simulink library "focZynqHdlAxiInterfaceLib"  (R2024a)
settings: Solver=VariableStepAuto  StartTime=0.0  StopTime=10.0  RelTol=1e-3
undefined symbols (not defined in the file or in its folder): AXI4, hex2dec, Lite
libraries: axiinterfacelib x14

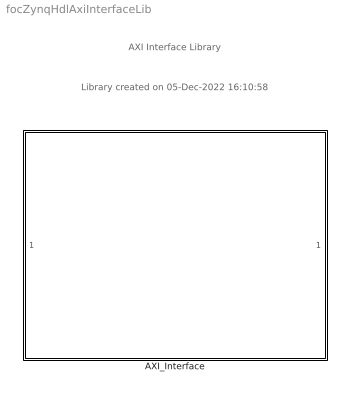
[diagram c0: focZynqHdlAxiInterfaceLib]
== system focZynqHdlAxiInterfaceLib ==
  note: AXI Interface Library
  note: Library created on 05-Dec-2022 16:10:58
  AXI_Interface : Subsystem  TreatAsAtomicUnit=on  mask(AXI4-Lite/AXI4 Interface){}
      mask help: This is an automatically generated subsystem block. This contains the AXI interface blocks that communicate with the focZynqHd_ip IPCore generated from focZynqHdl subsystem.

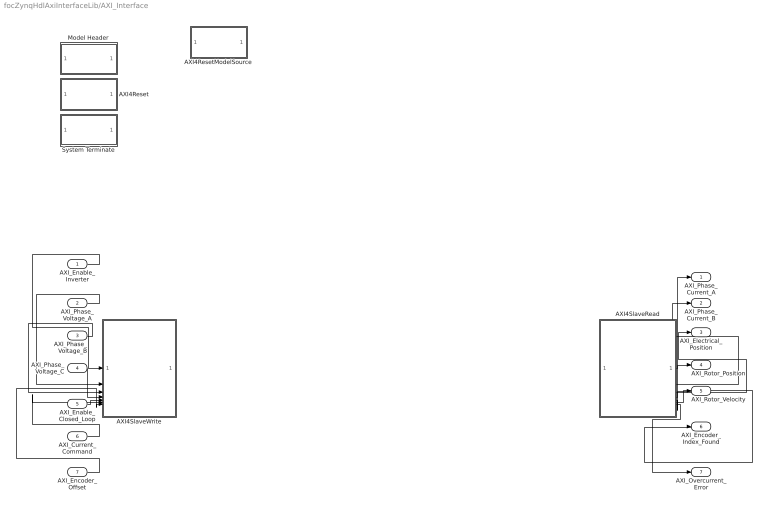
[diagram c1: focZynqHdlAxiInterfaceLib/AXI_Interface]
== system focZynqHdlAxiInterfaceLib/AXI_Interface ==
  AXI_Enable_Inverter : Inport
  AXI_Phase_Voltage_A : Inport  Port=2
  AXI_Phase_Voltage_B : Inport  Port=3
  AXI_Phase_Voltage_C : Inport  Port=4
  AXI_Enable_Closed_Loop : Inport  Port=5
  AXI_Current_Command : Inport  Port=6
  AXI_Encoder_Offset : Inport  Port=7
  AXI4Reset : Subsystem  mask(System Start){ShowInLibBrowser=0}
      mask prompts: ShowInLibBrowser "Simulink:masks:CustCodeMaskParam1_MP"
  AXI4ResetModelSource : Subsystem  mask(Model Source){ShowInLibBrowser=0}
      mask prompts: ShowInLibBrowser "Simulink:masks:CustCodeMaskParam1_MP"
  AXI4SlaveRead : Subsystem  Priority=10
  AXI4SlaveWrite : Subsystem  Priority=1
  Model Header : Subsystem  mask(Model Header){ShowInLibBrowser=0}
      mask prompts: ShowInLibBrowser "Simulink:masks:CustCodeMaskParam1_MP"
  System Terminate : Subsystem  mask(System Terminate){ShowInLibBrowser=0}
      mask prompts: ShowInLibBrowser "Simulink:masks:CustCodeMaskParam1_MP"
  AXI_Phase_Current_A : Outport  VectorParamsAs1DForOutWhenUnconnected=off
  AXI_Phase_Current_B : Outport  Port=2  VectorParamsAs1DForOutWhenUnconnected=off
  AXI_Electrical_Position : Outport  Port=3  VectorParamsAs1DForOutWhenUnconnected=off
  AXI_Rotor_Position : Outport  Port=4  VectorParamsAs1DForOutWhenUnconnected=off
  AXI_Rotor_Velocity : Outport  Port=5  VectorParamsAs1DForOutWhenUnconnected=off
  AXI_Encoder_Index_Found : Outport  Port=6  VectorParamsAs1DForOutWhenUnconnected=off
  AXI_Overcurrent_Error : Outport  Port=7  VectorParamsAs1DForOutWhenUnconnected=off
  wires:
  AXI4SlaveRead/7(AXI_Overcurrent_Error) -> AXI_Overcurrent_Error/1
  AXI4SlaveRead/6(AXI_Encoder_Index_Found) -> AXI_Encoder_Index_Found/1
  AXI4SlaveRead/5(AXI_Rotor_Velocity) -> AXI_Rotor_Velocity/1
  AXI4SlaveRead/4(AXI_Rotor_Position) -> AXI_Rotor_Position/1
  AXI4SlaveRead/3(AXI_Electrical_Position) -> AXI_Electrical_Position/1
  AXI4SlaveRead/2(AXI_Phase_Current_B) -> AXI_Phase_Current_B/1
  AXI4SlaveRead/1(AXI_Phase_Current_A) -> AXI_Phase_Current_A/1
  AXI_Encoder_Offset/1 -> AXI4SlaveWrite/7(AXI_Encoder_Offset)
  AXI_Current_Command/1 -> AXI4SlaveWrite/6(AXI_Current_Command)
  AXI_Enable_Closed_Loop/1 -> AXI4SlaveWrite/5(AXI_Enable_Closed_Loop)
  AXI_Phase_Voltage_C/1 -> AXI4SlaveWrite/4(AXI_Phase_Voltage_C)
  AXI_Phase_Voltage_B/1 -> AXI4SlaveWrite/3(AXI_Phase_Voltage_B)
  AXI_Phase_Voltage_A/1 -> AXI4SlaveWrite/2(AXI_Phase_Voltage_A)
  AXI_Enable_Inverter/1 -> AXI4SlaveWrite/1(AXI_Enable_Inverter)

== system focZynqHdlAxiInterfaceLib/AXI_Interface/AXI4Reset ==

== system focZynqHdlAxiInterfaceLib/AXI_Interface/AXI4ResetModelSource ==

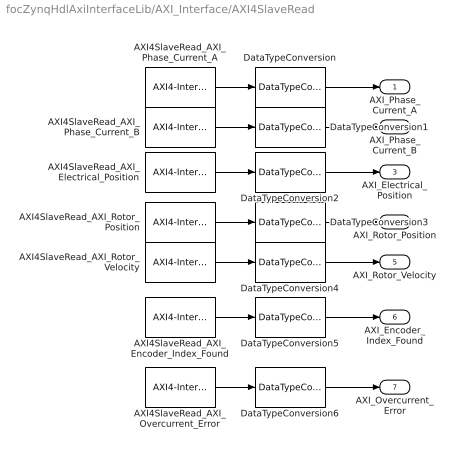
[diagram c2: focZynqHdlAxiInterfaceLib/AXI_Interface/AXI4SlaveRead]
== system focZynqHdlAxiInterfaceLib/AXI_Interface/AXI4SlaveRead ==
  AXI4SlaveRead_AXI_Electrical_Position : axiinterfacelib/AXI4-Interface Read  Priority=5  AXIInterfaceType=AXI4-Lite  DeviceName=/dev/mwipcore  RegisterOffset=hex2dec('124')  DataLength=1  DataType=uint32  SampleTime=-1  blockPlatform=ZYNQ  SimulateUsing=Interpreted Execution
  AXI4SlaveRead_AXI_Encoder_Index_Found : axiinterfacelib/AXI4-Interface Read  Priority=8  AXIInterfaceType=AXI4-Lite  DeviceName=/dev/mwipcore  RegisterOffset=hex2dec('130')  DataLength=1  DataType=uint32  SampleTime=-1  blockPlatform=ZYNQ  SimulateUsing=Interpreted Execution
  AXI4SlaveRead_AXI_Overcurrent_Error : axiinterfacelib/AXI4-Interface Read  Priority=9  AXIInterfaceType=AXI4-Lite  DeviceName=/dev/mwipcore  RegisterOffset=hex2dec('134')  DataLength=1  DataType=uint32  SampleTime=-1  blockPlatform=ZYNQ  SimulateUsing=Interpreted Execution
  AXI4SlaveRead_AXI_Phase_Current_A : axiinterfacelib/AXI4-Interface Read  Priority=3  AXIInterfaceType=AXI4-Lite  DeviceName=/dev/mwipcore  RegisterOffset=hex2dec('11C')  DataLength=1  DataType=uint32  SampleTime=-1  blockPlatform=ZYNQ  SimulateUsing=Interpreted Execution
  AXI4SlaveRead_AXI_Phase_Current_B : axiinterfacelib/AXI4-Interface Read  Priority=4  AXIInterfaceType=AXI4-Lite  DeviceName=/dev/mwipcore  RegisterOffset=hex2dec('120')  DataLength=1  DataType=uint32  SampleTime=-1  blockPlatform=ZYNQ  SimulateUsing=Interpreted Execution
  AXI4SlaveRead_AXI_Rotor_Position : axiinterfacelib/AXI4-Interface Read  Priority=6  AXIInterfaceType=AXI4-Lite  DeviceName=/dev/mwipcore  RegisterOffset=hex2dec('128')  DataLength=1  DataType=uint32  SampleTime=-1  blockPlatform=ZYNQ  SimulateUsing=Interpreted Execution
  AXI4SlaveRead_AXI_Rotor_Velocity : axiinterfacelib/AXI4-Interface Read  Priority=7  AXIInterfaceType=AXI4-Lite  DeviceName=/dev/mwipcore  RegisterOffset=hex2dec('12C')  DataLength=1  DataType=uint32  SampleTime=-1  blockPlatform=ZYNQ  SimulateUsing=Interpreted Execution
  DataTypeConversion : DataTypeConversion  OutDataTypeStr=fixdt(1,16,11)  ConvertRealWorld=Stored Integer (SI)
  DataTypeConversion1 : DataTypeConversion  OutDataTypeStr=fixdt(1,16,11)  ConvertRealWorld=Stored Integer (SI)
  DataTypeConversion2 : DataTypeConversion  OutDataTypeStr=fixdt(1,16,12)  ConvertRealWorld=Stored Integer (SI)
  DataTypeConversion3 : DataTypeConversion  OutDataTypeStr=fixdt(1,16,12)  ConvertRealWorld=Stored Integer (SI)
  DataTypeConversion4 : DataTypeConversion  OutDataTypeStr=fixdt(1,16,5)  ConvertRealWorld=Stored Integer (SI)
  DataTypeConversion5 : DataTypeConversion  OutDataTypeStr=fixdt('boolean')  ConvertRealWorld=Stored Integer (SI)
  DataTypeConversion6 : DataTypeConversion  OutDataTypeStr=fixdt('boolean')  ConvertRealWorld=Stored Integer (SI)
  AXI_Phase_Current_A : Outport  VectorParamsAs1DForOutWhenUnconnected=off
  AXI_Phase_Current_B : Outport  Port=2  VectorParamsAs1DForOutWhenUnconnected=off
  AXI_Electrical_Position : Outport  Port=3  VectorParamsAs1DForOutWhenUnconnected=off
  AXI_Rotor_Position : Outport  Port=4  VectorParamsAs1DForOutWhenUnconnected=off
  AXI_Rotor_Velocity : Outport  Port=5  VectorParamsAs1DForOutWhenUnconnected=off
  AXI_Encoder_Index_Found : Outport  Port=6  VectorParamsAs1DForOutWhenUnconnected=off
  AXI_Overcurrent_Error : Outport  Port=7  VectorParamsAs1DForOutWhenUnconnected=off
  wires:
  DataTypeConversion6/1 -> AXI_Overcurrent_Error/1
  AXI4SlaveRead_AXI_Overcurrent_Error/1 -> DataTypeConversion6/1
  DataTypeConversion4/1 -> AXI_Rotor_Velocity/1
  DataTypeConversion/1 -> AXI_Phase_Current_A/1
  DataTypeConversion5/1 -> AXI_Encoder_Index_Found/1
  AXI4SlaveRead_AXI_Encoder_Index_Found/1 -> DataTypeConversion5/1
  AXI4SlaveRead_AXI_Electrical_Position/1 -> DataTypeConversion2/1
  AXI4SlaveRead_AXI_Phase_Current_B/1 -> DataTypeConversion1/1
  DataTypeConversion2/1 -> AXI_Electrical_Position/1
  AXI4SlaveRead_AXI_Phase_Current_A/1 -> DataTypeConversion/1
  DataTypeConversion1/1 -> AXI_Phase_Current_B/1
  DataTypeConversion3/1 -> AXI_Rotor_Position/1
  AXI4SlaveRead_AXI_Rotor_Position/1 -> DataTypeConversion3/1
  AXI4SlaveRead_AXI_Rotor_Velocity/1 -> DataTypeConversion4/1

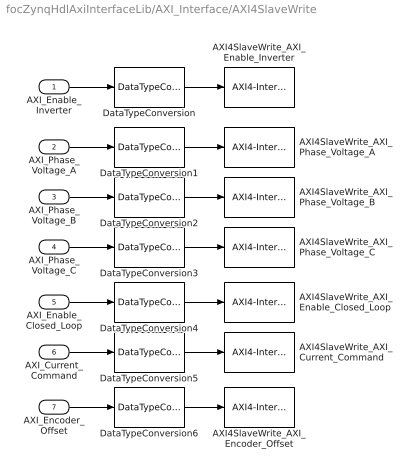
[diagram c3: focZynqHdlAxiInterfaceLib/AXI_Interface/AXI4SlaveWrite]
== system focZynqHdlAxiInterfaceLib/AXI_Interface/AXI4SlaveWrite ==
  AXI_Enable_Inverter : Inport
  AXI_Phase_Voltage_A : Inport  Port=2
  AXI_Phase_Voltage_B : Inport  Port=3
  AXI_Phase_Voltage_C : Inport  Port=4
  AXI_Enable_Closed_Loop : Inport  Port=5
  AXI_Current_Command : Inport  Port=6
  AXI_Encoder_Offset : Inport  Port=7
  AXI4SlaveWrite_AXI_Current_Command : axiinterfacelib/AXI4-Interface Write  Priority=7  AXIInterfaceType=AXI4-Lite  DeviceName=/dev/mwipcore  RegisterOffset=hex2dec('114')  blockPlatform=ZYNQ  SimulateUsing=Interpreted execution
  AXI4SlaveWrite_AXI_Enable_Closed_Loop : axiinterfacelib/AXI4-Interface Write  Priority=6  AXIInterfaceType=AXI4-Lite  DeviceName=/dev/mwipcore  RegisterOffset=hex2dec('110')  blockPlatform=ZYNQ  SimulateUsing=Interpreted execution
  AXI4SlaveWrite_AXI_Enable_Inverter : axiinterfacelib/AXI4-Interface Write  Priority=2  AXIInterfaceType=AXI4-Lite  DeviceName=/dev/mwipcore  RegisterOffset=hex2dec('100')  blockPlatform=ZYNQ  SimulateUsing=Interpreted execution
  AXI4SlaveWrite_AXI_Encoder_Offset : axiinterfacelib/AXI4-Interface Write  Priority=8  AXIInterfaceType=AXI4-Lite  DeviceName=/dev/mwipcore  RegisterOffset=hex2dec('118')  blockPlatform=ZYNQ  SimulateUsing=Interpreted execution
  AXI4SlaveWrite_AXI_Phase_Voltage_A : axiinterfacelib/AXI4-Interface Write  Priority=3  AXIInterfaceType=AXI4-Lite  DeviceName=/dev/mwipcore  RegisterOffset=hex2dec('104')  blockPlatform=ZYNQ  SimulateUsing=Interpreted execution
  AXI4SlaveWrite_AXI_Phase_Voltage_B : axiinterfacelib/AXI4-Interface Write  Priority=4  AXIInterfaceType=AXI4-Lite  DeviceName=/dev/mwipcore  RegisterOffset=hex2dec('108')  blockPlatform=ZYNQ  SimulateUsing=Interpreted execution
  AXI4SlaveWrite_AXI_Phase_Voltage_C : axiinterfacelib/AXI4-Interface Write  Priority=5  AXIInterfaceType=AXI4-Lite  DeviceName=/dev/mwipcore  RegisterOffset=hex2dec('10C')  blockPlatform=ZYNQ  SimulateUsing=Interpreted execution
  DataTypeConversion{,1..6} (7 alike) : DataTypeConversion  OutDataTypeStr=fixdt(0,32,0)  ConvertRealWorld=Stored Integer (SI)
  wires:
  DataTypeConversion3/1 -> AXI4SlaveWrite_AXI_Phase_Voltage_C/1
  AXI_Phase_Voltage_C/1 -> DataTypeConversion3/1
  AXI_Current_Command/1 -> DataTypeConversion5/1
  DataTypeConversion1/1 -> AXI4SlaveWrite_AXI_Phase_Voltage_A/1
  DataTypeConversion/1 -> AXI4SlaveWrite_AXI_Enable_Inverter/1
  AXI_Encoder_Offset/1 -> DataTypeConversion6/1
  DataTypeConversion6/1 -> AXI4SlaveWrite_AXI_Encoder_Offset/1
  AXI_Enable_Closed_Loop/1 -> DataTypeConversion4/1
  AXI_Phase_Voltage_B/1 -> DataTypeConversion2/1
  DataTypeConversion4/1 -> AXI4SlaveWrite_AXI_Enable_Closed_Loop/1
  DataTypeConversion2/1 -> AXI4SlaveWrite_AXI_Phase_Voltage_B/1
  DataTypeConversion5/1 -> AXI4SlaveWrite_AXI_Current_Command/1
  AXI_Phase_Voltage_A/1 -> DataTypeConversion1/1
  AXI_Enable_Inverter/1 -> DataTypeConversion/1

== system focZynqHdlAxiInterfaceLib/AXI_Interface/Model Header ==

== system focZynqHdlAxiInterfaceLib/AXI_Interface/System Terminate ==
